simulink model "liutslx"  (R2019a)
settings: configuration reference "configurationSettings" (kept in a data dictionary, not in this file)
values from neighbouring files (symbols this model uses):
  L = fbtc(P,G)    [fbt.m]    (also in fbtc.m = meqc(P,G,'rrx','zzx'); fbte.m = varargout{1}; fge.m = fgel(L,meqxk(LX,1)); fgec.m = fgsc(P,G))
libraries: liulib x1

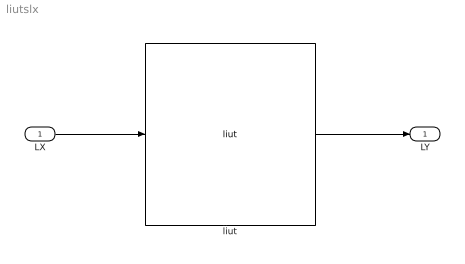
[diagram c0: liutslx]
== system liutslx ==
  LX : Inport  OutDataTypeStr=Bus: LXbus  PortDimensions=1  SampleTime=L.dt  Interpolate=off
  liut : liulib/liut  SystemSampleTime=-1
  LY : Outport  OutDataTypeStr=Bus: LYbus  PortDimensions=1
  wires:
  LX/1 -> liut/1
  liut/1 -> LY/1
